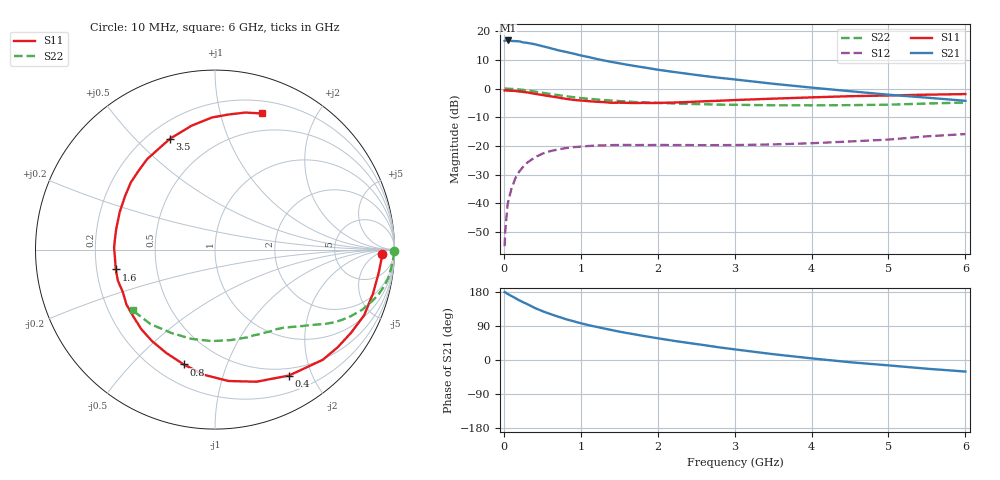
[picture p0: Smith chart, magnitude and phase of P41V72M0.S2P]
! SIEMENS Small Signal Semiconductors
! BFP182
! Si NPN RF Bipolar Junction Transistor in SOT143
! VCE = 1.75 V  IC = 2 mA
! Common Emitter S-Parameters:  March  1996
# GHz  S  MA  R  50
!  f  S11  S21  S12  S22
! GHz  MAG  ANG  MAG  ANG  MAG  ANG  MAG  ANG
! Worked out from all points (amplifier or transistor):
!   36 points, 10 MHz to 6 GHz, reference 50 ohm
!   highest |S21| = 16.8 dB at 50 MHz (marker M1)
!   |S21| within 3 dB of that: start of sweep to 648.7 MHz
!   unconditionally stable (mu >= 1): 2.16 GHz to end of sweep
!   at 250 MHz: K = 0.12, MSG = 21.7 dB, |S12| = -27.3 dB
!   at 1.4 GHz: K = 0.68, MSG = 14.5 dB, |S12| = -19.7 dB
!   at 6 GHz: K = 1.01, MAG = 5.2 dB, |S12| = -15.9 dB
!   S11 on the Smith chart (normalised r, x): 10 MHz: 24, -9; 400 MHz: 0.40, -1.67; 800 MHz: 0.31, -0.72; 1.6 GHz: 0.28, -0.09; 3.5 GHz: 0.29, +0.63; 6 GHz: 0.32, +1.35
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0.01  0.9289 -1.6  6.774 179.2  0.0018 91.0  0.9968 -0.6
0.02  0.929 -3.2  6.854 178.4  0.0035 82.0  0.9971 -1.2
0.05  0.921 -8.1  6.879 174.4  0.0099 85.7  0.9941 -3.1
0.1  0.9138 -15.5  6.736 168.8  0.0181 79.6  0.9863 -6.2
0.2  0.8885 -31.4  6.638 157.6  0.0358 72.1  0.9645 -12.2
0.25  0.8738 -38.5  6.372 152.5  0.0433 68.0  0.9469 -15.0
0.3  0.8587 -45.7  6.257 147.9  0.0507 63.8  0.928 -17.4
0.4  0.8137 -59.6  5.917 137.6  0.063 56.4  0.8871 -22.1
0.5  0.7714 -72.6  5.473 129.0  0.0734 50.1  0.8442 -26.0
0.6  0.736 -84.1  5.075 121.6  0.0811 44.5  0.8059 -29.2
0.8  0.6631 -105.2  4.367 108.2  0.0916 35.6  0.7378 -34.2
1  0.6189 -124.6  3.773 97.1  0.0974 28.8  0.6838 -37.9
1.1  0.6042 -132.8  3.538 91.9  0.1 26.2  0.6635 -39.6
1.3  0.5807 -148.1  3.088 83.3  0.1026 21.7  0.6313 -42.5
1.6  0.5637 -168.7  2.604 71.2  0.1043 17.1  0.5957 -46.6
1.8  0.5623 178.7  2.357 64.0  0.104 15.7  0.576 -49.2
2.2  0.5706 158.5  1.954 50.9  0.1037 12.9  0.5519 -55.3
2.8  0.6128 133.6  1.54 33.3  0.1034 12.1  0.5246 -65.6
3.5  0.6668 112.1  1.212 15.4  0.1064 13.2  0.5117 -80.1
4.5  0.7361 91.4  0.899 -5.9  0.1199 15.7  0.5143 -104.7
5.5  0.7821 77.5  0.694 -23.0  0.1473 16.2  0.5488 -130.8
6  0.8017 71.1  0.612 -30.5  0.1611 13.2  0.5701 -143.5
